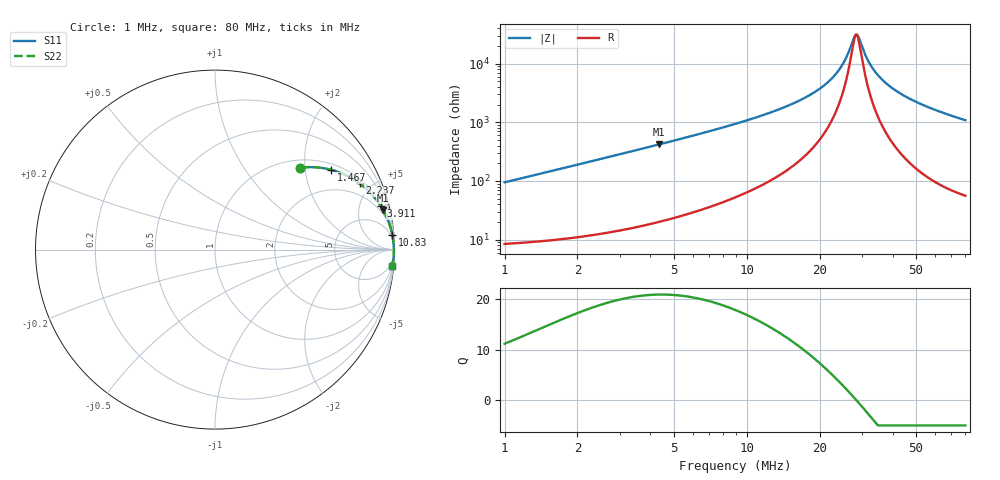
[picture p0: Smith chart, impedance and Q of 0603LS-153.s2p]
# MHz S MA R 50
!Freq  MagS11  AngS11  MagS21  AngS21  MagS12  AngS12  MagS22  AngS22
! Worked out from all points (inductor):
!   801 points, 1 MHz to 80 MHz, reference 50 ohm
!   read as one part in series: L = 15 uH near 1.022 MHz
!   highest Q = 20.9 at 4.34 MHz (marker M1), where L = 15.3 uH
!   self-resonance near 28.26 MHz
!   S11 on the Smith chart (normalised r, x): 1 MHz: 1.17, +1.89; 1.467 MHz: 1.19, +2.77; 2.237 MHz: 1.23, +4.24; 3.911 MHz: 1.36, +7.51; 10.83 MHz: 2, +24; 80 MHz: 2, -22
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1  0.6589 43.9  0.6956 -41.0  0.6956 -41.0  0.6589 43.9
1.467305  0.7864 34.4  0.566 -51.7  0.566 -51.7  0.7864 34.4
2.237138  0.8861 24.6  0.4172 -62.2  0.4172 -62.2  0.8861 24.6
3.911441  0.955 14.7  0.2541 -72.5  0.2541 -72.5  0.955 14.7
4.340454  0.9623 13.3  0.2297 -74.0  0.2297 -74.0  0.9623 13.3
7.028701  0.9831 8.0  0.1393 -79.1  0.1393 -79.1  0.9831 8.0
10.83441  0.9914 4.8  0.08302 -81.7  0.08302 -81.7  0.9914 4.8
14.16999  0.9941 3.2  0.05599 -82.3  0.05599 -82.3  0.9941 3.2
19.36264  0.9959 1.7  0.02935 -81.1  0.02935 -81.1  0.9959 1.7
22.82078  0.9964 0.9  0.01667 -77.2  0.01667 -77.2  0.9964 0.9
25.18547  0.9967 0.5  0.00946 -69.1  0.00946 -69.1  0.9967 0.5
27.34217  0.9968 0.2  0.004214 -40.1  0.004214 -40.1  0.9968 0.2
28.10135  0.9968 0.0  0.003265 -12.0  0.003265 -12.0  0.9968 0.0
28.72385  0.9968 -0.1  0.003316 16.7  0.003316 16.7  0.9968 -0.1
31.18356  0.9969 -0.4  0.007748 65.8  0.007748 65.8  0.9969 -0.4
33.30213  0.9968 -0.7  0.01242 74.9  0.01242 74.9  0.9968 -0.7
36.35246  0.9968 -1.1  0.01895 79.6  0.01895 79.6  0.9968 -1.1
40.56122  0.9965 -1.6  0.02742 82.0  0.02742 82.0  0.9965 -1.6
46.51388  0.9961 -2.2  0.03851 83.1  0.03851 83.1  0.9961 -2.2
53.9277  0.9953 -2.9  0.05131 83.3  0.05131 83.3  0.9953 -2.9
67.13769  0.9934 -4.1  0.07234 82.7  0.07234 82.7  0.9934 -4.1
80  0.9911 -5.2  0.09148 81.8  0.09148 81.8  0.9911 -5.2
